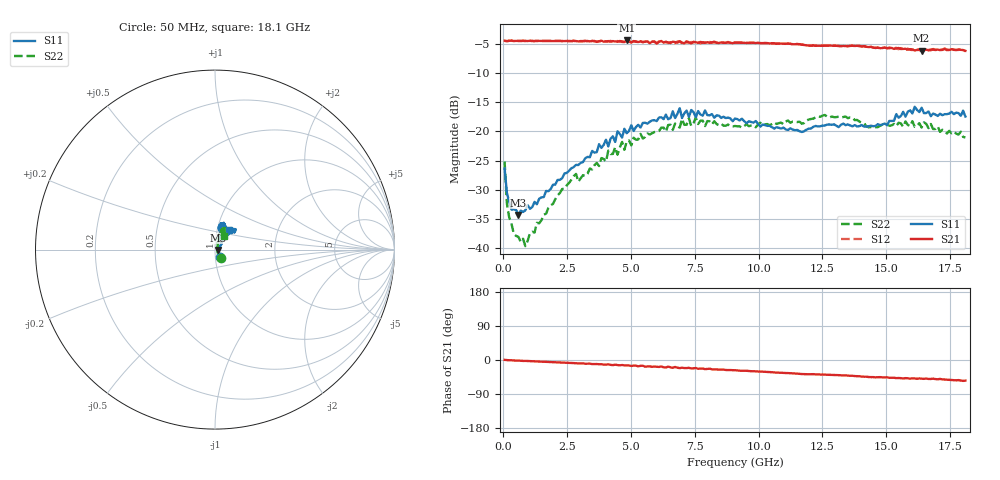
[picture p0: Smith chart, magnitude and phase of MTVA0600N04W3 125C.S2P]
! Network Analyzer HP8720D.06.14 Serial No. US36140669
!  8 Jul 2005  11:54:25
! Frequency  S11  S21  S12  S22
# HZ  S  DB R 50
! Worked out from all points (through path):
!   201 points, 50 MHz to 18.1 GHz, reference 50 ohm
!   highest |S21| = -4.48 dB at 4.833 GHz (marker M1); lowest = -6.2 dB at 16.39 GHz (marker M2)
!   group delay of S21, straight-line fit = 8.51 ps
!   lowest |S11| = -34.3 dB at 591.5 MHz (marker M3), VSWR 1.04, Z = 52 - j0.145 ohm
!   |S11| at or under -10 dB: start of sweep to end of sweep
!   |S22| runs from -39.6 to -17.2 dB; largest |S21 - S12| = 0.024
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5e7  -26.35 -56.8  -4.52 0.4  -4.55 0.4  -25.13 -54.7
1.4025e8  -30.54 -39.8  -4.61 -0.2  -4.58 -0.3  -32.34 -50.5
2.305e8  -32.03 -27.3  -4.54 -0.7  -4.52 -0.7  -34.71 -43.2
5.915e8  -34.29 -4.1  -4.53 -1.4  -4.58 -1.6  -38.02 -3.5
8.6225e8  -33.48 7.2  -4.55 -2.3  -4.58 -2.5  -39.60 19.1
2.30625e9  -27.98 36.7  -4.58 -6.8  -4.58 -6.9  -29.84 60.6
3.1185e9  -25.25 50.0  -4.58 -8.9  -4.61 -9.2  -27.50 70.8
4.021e9  -21.43 57.5  -4.63 -12.3  -4.64 -11.6  -25.17 70.8
4.11125e9  -22.57 57.6  -4.59 -11.5  -4.65 -12.5  -23.29 71.0
4.47225e9  -19.98 56.0  -4.70 -13.4  -4.57 -12.8  -23.99 76.5
4.83325e9  -20.31 66.5  -4.48 -14.3  -4.63 -14.9  -21.69 66.7
6.09675e9  -17.65 65.8  -4.72 -18.3  -4.63 -18.3  -19.94 70.3
6.7285e9  -17.73 73.3  -4.76 -18.4  -4.95 -19.2  -18.66 66.8
6.909e9  -16.05 72.0  -4.60 -21.5  -4.69 -20.2  -19.36 66.2
6.99925e9  -17.72 71.8  -4.84 -20.2  -4.95 -21.7  -17.88 67.9
7.36025e9  -16.35 68.8  -4.97 -22.3  -4.74 -21.6  -19.09 71.9
7.54075e9  -17.60 71.0  -4.79 -21.2  -4.68 -23.4  -17.66 70.9
9.075e9  -17.81 78.6  -4.85 -27.2  -4.82 -27.3  -19.08 61.5
1.21435e10  -19.22 67.5  -5.35 -37.4  -5.30 -37.6  -17.83 62.8
1.512175e10  -18.22 50.6  -5.79 -47.0  -5.67 -46.6  -19.05 64.2
1.638525e10  -15.96 43.7  -6.25 -49.1  -6.01 -48.8  -19.35 58.9
1.81e10  -17.46 55.8  -6.24 -54.3  -6.33 -55.2  -21.05 57.2
